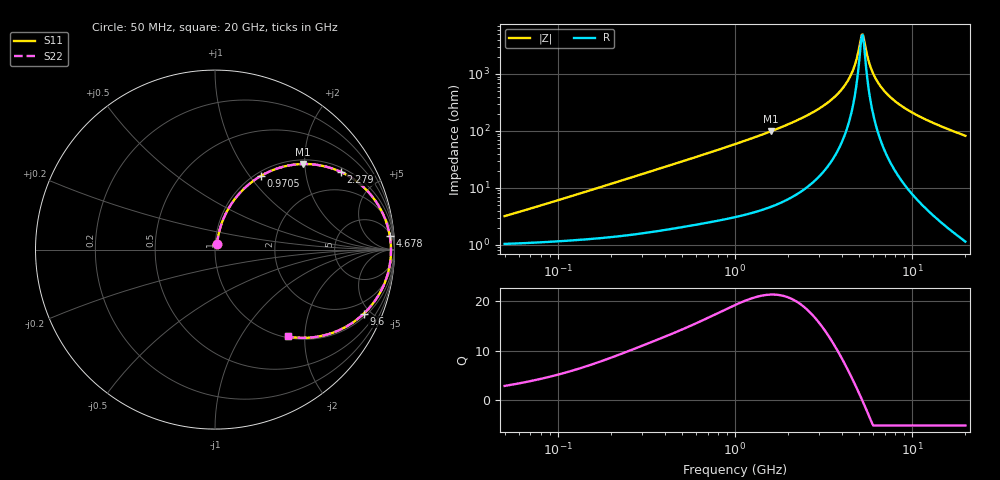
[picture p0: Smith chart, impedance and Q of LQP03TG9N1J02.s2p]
!Murata Part Number: LQP03TG9N1J02
!These Parameters are Measured in Series Mode Connection
!  o--[Z]--o
!Port1  Port2
!  o-------o
!Freq. Start=50[MHz] Stop=20[GHz], 401[Steps]
# Hz S RI R 50
!Freq.(Hz) S11(Real) S11(Imag) S21(Real) S21(Imag) S12(Real) S12(Imag) S22(Real) S22(Imag)
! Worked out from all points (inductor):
!   401 points, 50 MHz to 20 GHz, reference 50 ohm
!   read as one part in series: L = 9.56 nH near 52.3 MHz
!   highest Q = 21.2 at 1.591 GHz (marker M1), where L = 9.82 nH
!   self-resonance near 5.195 GHz
!   S11 on the Smith chart (normalised r, x): 50 MHz: 1.02, +0.06; 970.5 MHz: 1.06, +1.13; 2.279 GHz: 1.16, +3.14; 4.678 GHz: 7, +24; 9.6 GHz: 1.18, -4.53; 20 GHz: 1.02, -1.64
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5e7  0.0112 0.0296  0.9888 -0.0296  0.9888 -0.0296  0.0112 0.0296
1.364002e8  0.0184 0.0782  0.9816 -0.0782  0.9816 -0.0782  0.0184 0.0782
3.721004e8  0.0595 0.1994  0.9405 -0.1994  0.9405 -0.1994  0.0595 0.1994
6.285508e8  0.1318 0.308  0.8682 -0.308  0.8682 -0.308  0.1318 0.308
9.70487e8  0.2547 0.41  0.7453 -0.41  0.7453 -0.41  0.2547 0.41
1e9  0.2661 0.4165  0.7339 -0.4165  0.7339 -0.4165  0.2661 0.4165
1.590961e9  0.4917 0.4769  0.5083 -0.4769  0.5083 -0.4769  0.4917 0.4769
2.279204e9  0.7025 0.4323  0.2975 -0.4323  0.2975 -0.4323  0.7025 0.4323
2.728004e9  0.8002 0.3718  0.1998 -0.3718  0.1998 -0.3718  0.8002 0.3718
3.850025e9  0.9372 0.1959  0.0628 -0.1959  0.0628 -0.1959  0.9372 0.1959
4.34015e9  0.9639 0.1219  0.0361 -0.1219  0.0361 -0.1219  0.9639 0.1219
4.677679e9  0.9743 0.0739  0.0257 -0.0739  0.0257 -0.0739  0.9743 0.0739
5.117541e9  0.9803 0.0151  0.0197 -0.0151  0.0197 -0.0151  0.9803 0.0151
5.273168e9  0.9807 -0.00455  0.0193 0.00455  0.0193 0.00455  0.9807 -0.00455
5.352748e9  0.9806 -0.0144  0.0194 0.0144  0.0194 0.0144  0.9806 -0.0144
5.769027e9  0.977 -0.0636  0.023 0.0636  0.023 0.0636  0.977 -0.0636
6.034176e9  0.9725 -0.0928  0.0275 0.0928  0.0275 0.0928  0.9725 -0.0928
6.601595e9  0.9581 -0.1504  0.0419 0.1504  0.0419 0.1504  0.9581 -0.1504
7.442007e9  0.9282 -0.2237  0.0718 0.2237  0.0718 0.2237  0.9282 -0.2237
9.600142e9  0.8276 -0.3583  0.1724 0.3583  0.1724 0.3583  0.8276 -0.3583
1.375312e10  0.626 -0.4729  0.374 0.4729  0.374 0.4729  0.626 -0.4729
2e10  0.4042 -0.4839  0.5958 0.4839  0.5958 0.4839  0.4042 -0.4839
